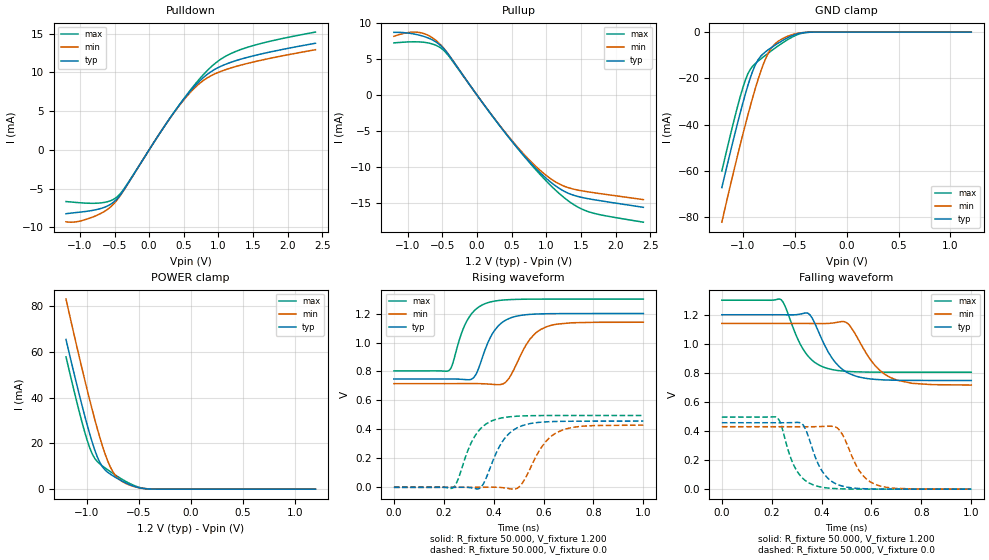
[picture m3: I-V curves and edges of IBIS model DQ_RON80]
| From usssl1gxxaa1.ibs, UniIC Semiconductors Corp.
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|   Model DQ_RON80
[Model] DQ_RON80
Model_type I/O
Vinl =  0.500V
Vinh =  0.700V
Vmeas =  0.600V
Rref =  50.000
Vref =  0.600V
C_comp   1.373pF   1.353pF   1.403pF
[Model Spec]
Vinh   0.700V   0.670V   0.750V
Vinl   0.500V   0.470V   0.550V
Vmeas   0.600V   0.570V   0.650V
Vref   0.600V   0.570V   0.650V
Rref   50.000   NA   NA
[Temperature Range]   25.000   0.125k   -40.000
[Voltage Range]   1.200V   1.140V   1.300V
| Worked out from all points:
|   slope of the pulldown table from 0 to 0.18 V, typ, clamps not added: 71.9 ohm
|   slope of the pullup table from 0 to 0.18 V, typ, clamps not added: 75.3 ohm
|   GND clamp passes 1 mA (typ) near -0.49 V on its own axis
|   POWER clamp passes 1 mA (typ) near -0.53 V on its own axis
|   rising waveform, R_fixture 50.000, V_fixture 1.200: 20-80 % time 72.8ps typ, 85.1ps min, 68.7ps max; typ from 0.748 V to 1.2 V
|   rising waveform, R_fixture 50.000, V_fixture 0.0: 20-80 % time 82.2ps typ, 90.6ps min, 76.9ps max; typ from 0 V to 0.457 V
|   falling waveform, R_fixture 50.000, V_fixture 1.200: 20-80 % time 92.9ps typ, 106ps min, 85.5ps max; typ from 1.2 V to 0.748 V
|   falling waveform, R_fixture 50.000, V_fixture 0.0: 20-80 % time 70.2ps typ, 77.4ps min, 66.2ps max; typ from 0.457 V to 0 V
[Pulldown]
|Voltage   I(typ)   I(min)   I(max)
-1.2V     -8.251mA   -9.292mA   -6.679mA
-1.015V   -8.058mA   -9.228mA   -6.82mA
-756mV    -7.708mA   -8.461mA   -6.891mA
-571mV    -7.108mA   -7.482mA   -6.618mA
-460mV    -6.305mA   -6.44mA    -6.057mA
-349mV    -4.95mA    -4.993mA   -4.856mA
354mV     4.778mA    4.742mA    4.779mA
613mV     7.774mA    7.594mA    7.918mA
798mV     9.448mA    9.048mA    9.855mA
1.02V     10.72mA    10.08mA    11.61mA
1.279V    11.59mA    10.83mA    12.8mA
2.4V      13.76mA    12.92mA    15.2mA
[Pullup]
|Voltage   I(typ)   I(min)   I(max)
-1.2V     8.762mA    8.211mA    7.299mA
-1.004V   8.671mA    8.724mA    7.423mA
-819mV    8.337mA    8.723mA    7.423mA
-634mV    7.655mA    7.934mA    7.109mA
-486mV    6.537mA    6.608mA    6.29mA
106mV     -1.418mA   -1.408mA   -1.399mA
513mV     -6.548mA   -6.441mA   -6.547mA
846mV     -10.2mA    -9.918mA   -10.39mA
1.142V    -12.72mA   -12.15mA   -13.34mA
1.364V    -13.86mA   -13.04mA   -15.07mA
1.586V    -14.41mA   -13.46mA   -16.18mA
2.4V      -15.65mA   -14.57mA   -17.72mA
[GND_clamp]
|Voltage   I(typ)   I(min)   I(max)
-1.2V     -67.26mA   -82.22mA   -60.1mA
-1.05V    -39.62mA   -53.62mA   -32.4mA
-1V       -31.05mA   -44.64mA   -24.37mA
-950mV    -23.16mA   -36.01mA   -18.1mA
-925mV    -19.62mA   -31.85mA   -16.02mA
-875mV    -13.89mA   -23.97mA   -13.48mA
-800mV    -9.288mA   -13.81mA   -10.72mA
-750mV    -7.535mA   -8.829mA   -8.993mA
-675mV    -5.274mA   -4.578mA   -6.506mA
-525mV    -1.587mA   -1.138mA   -2.208mA
-375mV    -90.13uA   -87.27uA   -132.9uA
1.2V      0A         0A         0A
[POWER_clamp]
|Voltage   I(typ)   I(min)   I(max)
-1.2V     65.51mA    83.21mA    57.91mA
-1.05V    37.38mA    53.57mA    29.99mA
-1V       28.74mA    44.18mA    21.95mA
-950mV    20.85mA    35.16mA    15.65mA
-925mV    17.34mA    30.84mA    13.56mA
-875mV    11.74mA    22.7mA     11.06mA
-800mV    7.436mA    12.47mA    8.502mA
-750mV    5.864mA    7.69mA     6.933mA
-675mV    3.901mA    3.837mA    4.735mA
-525mV    971.5uA    903.1uA    1.25mA
-400mV    85.95uA    125.9uA    91.19uA
1.2V      0A         0A         0A
[Ramp]
| variable   typ   min   max
dV/dt_r   0.274/82.196p   0.258/90.821p   0.298/77.431p
dV/dt_f   0.271/93.267p   0.254/0.106n   0.297/85.719p
R_load = 50.000
[Rising Waveform]
R_fixture= 50.000
V_fixture= 1.200
V_fixture_min= 1.140
V_fixture_max= 1.300
|time   V(typ)   V(min)   V(max)
0s        747.7mV    716mV      804.3mV
221ps     748mV      716mV      806.7mV
236ps     747.9mV    716mV      855.6mV
278ps     745.1mV    716.2mV    1.096V
319ps     756mV      716.4mV    1.214V
378ps     1.004V     713.2mV    1.276V
451ps     1.157V     731.1mV    1.295V
546ps     1.194V     1.024V     1.299V
615ps     1.199V     1.111V     1.3V
1ns       1.2V       1.14V      1.3V
[Rising Waveform]
R_fixture= 50.000
V_fixture= 0.0
V_fixture_min= 0.0
V_fixture_max= 0.0
|time   V(typ)   V(min)   V(max)
0s        53.9nV     938.4nV    31.31nV
237ps     78.98uV    -5.116uV   -3.156mV
307ps     -2.325mV   -17.38uV   297.5mV
349ps     214.9uV    236.1uV    407.7mV
414ps     251.8mV    389.6uV    471.8mV
453ps     356.4mV    -6.442mV   484.8mV
502ps     417.4mV    2.434mV    491.9mV
585ps     449mV      259.9mV    495.4mV
654ps     454.9mV    379.6mV    496mV
1ns       457mV      429.6mV    496.2mV
[Falling Waveform]
R_fixture= 50.000
V_fixture= 1.200
V_fixture_min= 1.140
V_fixture_max= 1.300
|time   V(typ)   V(min)   V(max)
0s        1.2V       1.14V      1.3V
238ps     1.2V       1.14V      1.303V
304ps     1.201V     1.14V      1.034V
347ps     1.209V     1.14V      913.2mV
426ps     944.9mV    1.14V      829.5mV
504ps     801.4mV    1.141V     810.2mV
596ps     758.2mV    890.1mV    805.3mV
675ps     750.3mV    768.7mV    804.5mV
764ps     748.2mV    728.1mV    804.3mV
1ns       747.7mV    716.2mV    804.3mV
[Falling Waveform]
R_fixture= 50.000
V_fixture= 0.0
V_fixture_min= 0.0
V_fixture_max= 0.0
|time   V(typ)   V(min)   V(max)
0s        457mV      429.7mV    496.2mV
221ps     456.9mV    429.7mV    493.4mV
281ps     457.9mV    429.6mV    193.5mV
322ps     448.6mV    429.4mV    78.83mV
380ps     197.8mV    430.1mV    21.58mV
424ps     76.52mV    432.8mV    8.102mV
467ps     29.75mV    414.9mV    3.09mV
551ps     4.614mV    126.7mV    470.6uV
614ps     1.151mV    33.43mV    115.2uV
1ns       263.1nV    8.522uV    45.07nV
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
